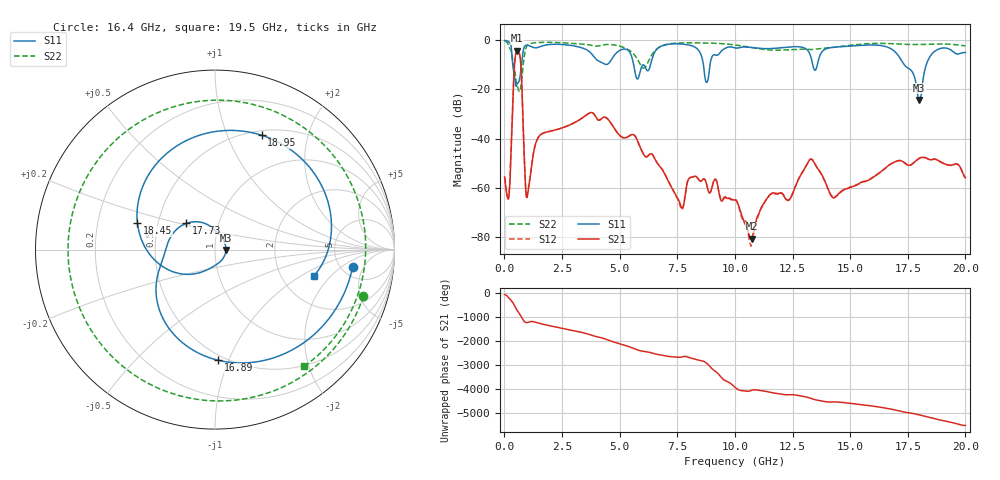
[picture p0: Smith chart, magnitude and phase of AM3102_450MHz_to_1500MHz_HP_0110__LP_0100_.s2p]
!Agilent Technologies,E8364B,MY43040894,A.07.50.67
!Agilent E8364B: A.07.50.67
!Date: Thursday, January 11, 2018 05:46:40
!Correction: S11(Full 2 Port(1,2))
!S21(Full 2 Port(1,2))
!S12(Full 2 Port(1,2))
!S22(Full 2 Port(1,2))
!S2P File: Measurements: S11, S21, S12, S22:
# Hz S  dB  R 50
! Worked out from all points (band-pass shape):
!   1601 points, 10 MHz to 20 GHz, reference 50 ohm
!   highest |S21| = -4.28 dB at 559.7 MHz (marker M1); lowest = -80.7 dB at 10.73 GHz (marker M2)
!   |S21| within 3 dB of the highest: 465.5 MHz to 688 MHz (222.4 MHz wide, 38.6 % of centre)
!   lowest |S11| = -24.3 dB at 18 GHz (marker M3), VSWR 1.13, Z = 56.5 - j0.24 ohm
!   |S11| at or under -10 dB: 364 MHz to 741.2 MHz (377.2 MHz wide, 68.3 % of centre); 5.608 GHz to 6.008 GHz (400 MHz wide, 6.89 % of centre); 17.35 GHz to 18.3 GHz (948.9 MHz wide, 5.32 % of centre)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
!   |S22| runs from -20.8 to -0.3 dB; largest |S21 - S12| = 0.0022
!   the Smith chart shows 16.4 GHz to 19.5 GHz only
!   S11 on the Smith chart (normalised r, x): 16.4 GHz: 6.28, -3.06; 16.89 GHz: 0.46, -0.92; 17.73 GHz: 0.70, +0.21; 18.45 GHz: 0.38, +0.14; 18.95 GHz: 0.55, +1.34; 19.5 GHz: 3.04, -1.31
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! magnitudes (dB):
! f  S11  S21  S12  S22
! 10 MHz  -0.1  -55.6  -55.8  -0.3
! 197.4 MHz  -0.7  -63.4  -62.6  -2.5
! 559.7 MHz  -17.4  -4.3  -4.3  -18.8
! 997 MHz  -2.0  -63.2  -63.2  -2.1
! 1.509 GHz  -2.7  -39.0  -39.0  -0.9
! 3.346 GHz  -3.0  -31.8  -31.8  -1.5
! 6.682 GHz  -3.0  -50.5  -50.5  -3.0
! 7.681 GHz  -1.5  -67.9  -68.7  -1.1
! 8.781 GHz  -17.1  -58.9  -58.9  -1.1
! 10.01 GHz  -3.1  -64.9  -64.9  -1.9
! 10.73 GHz  -3.0  -80.7  -82.5  -3.0
! 13.34 GHz  -8.4  -48.4  -48.4  -3.8
! 14.28 GHz  -2.8  -64.1  -63.8  -2.9
! 16.4 GHz  -2.2  -52.9  -53.0  -1.2
! 16.68 GHz  -3.0  -50.8  -50.9  -1.3
! 16.89 GHz  -4.2  -49.6  -49.7  -1.4
! 17.73 GHz  -13.3  -50.1  -50.0  -1.7
! 18 GHz  -24.3  -48.0  -48.0  -1.7
! 18.45 GHz  -6.8  -48.6  -48.5  -1.6
! 18.95 GHz  -3.2  -49.5  -49.7  -1.5
! 19.5 GHz  -4.9  -50.5  -50.5  -1.7
! 20 GHz  -5.0  -55.9  -56.0  -2.3
